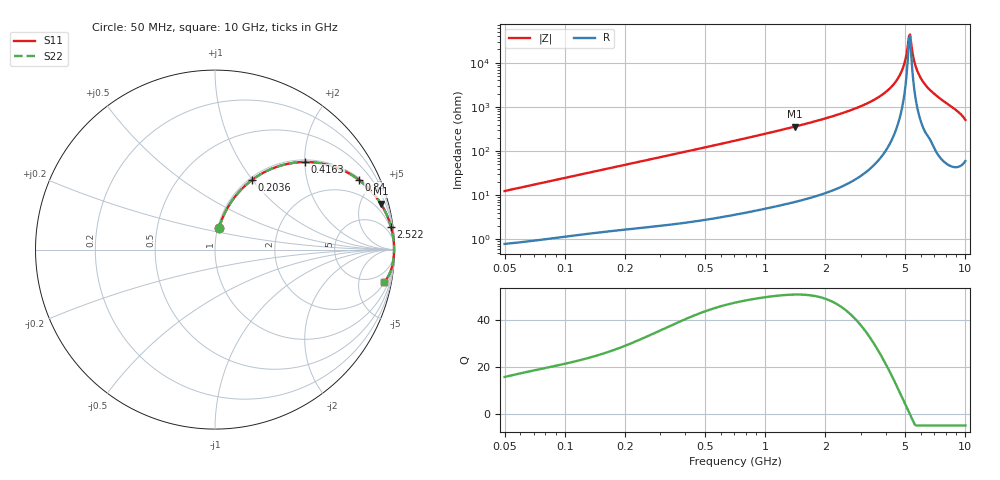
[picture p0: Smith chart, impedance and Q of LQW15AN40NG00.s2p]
!Murata Part Number: LQW15AN40NG00
!These Parameters are Measured in Series Mode Connection
!  o--[Z]--o
!Port1  Port2
!  o-------o
!Freq. Start=50[MHz] Stop=10[GHz], 401[Steps]
# Hz S RI R 50
!Freq.(Hz)	S 11(Real)	S 11(Imag)	S 21(Real)	S 21(Imag)	S 12(Real)	S 12(Imag)	S 22(Real)	S 22(Imag)
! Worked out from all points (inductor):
!   401 points, 50 MHz to 10 GHz, reference 50 ohm
!   read as one part in series: L = 39.4 nH near 51.34 MHz
!   highest Q = 51 at 1.408 GHz (marker M1), where L = 40.5 nH
!   self-resonance near 5.225 GHz
!   S11 on the Smith chart (normalised r, x): 50 MHz: 1.02, +0.25; 203.6 MHz: 1.03, +0.99; 416.3 MHz: 1.05, +2.01; 840 MHz: 1.08, +4.10; 2.522 GHz: 1, +15; 10 GHz: 2, -10
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5e7  0.0227 0.1205  0.9773 -0.1205  0.9773 -0.1205  0.0227 0.1205
1.214486e8  0.0909 0.2666  0.9091 -0.2666  0.9091 -0.2666  0.0909 0.2666
2.035837e8  0.2039 0.3862  0.7961 -0.3862  0.7961 -0.3862  0.2039 0.3862
2.949953e8  0.3409 0.4601  0.6591 -0.4601  0.6591 -0.4601  0.3409 0.4601
4.162766e8  0.5022 0.488  0.4978 -0.488  0.4978 -0.488  0.5022 0.488
7.071068e8  0.7424 0.4269  0.2576 -0.4269  0.2576 -0.4269  0.7424 0.4269
8.399791e8  0.8032 0.3875  0.1968 -0.3875  0.1968 -0.3875  0.8032 0.3875
1.408053e9  0.9235 0.2561  0.0765 -0.2561  0.0765 -0.2561  0.9235 0.2561
1.717543e9  0.9498 0.2087  0.0502 -0.2087  0.0502 -0.2087  0.9498 0.2087
2.521925e9  0.9805 0.1276  0.0195 -0.1276  0.0195 -0.1276  0.9805 0.1276
3.420121e9  0.9924 0.0722  0.00758 -0.0722  0.00758 -0.0722  0.9924 0.0722
4.171863e9  0.9964 0.0387  0.00363 -0.0387  0.00363 -0.0387  0.9964 0.0387
4.762728e9  0.9976 0.0168  0.00236 -0.0168  0.00236 -0.0168  0.9976 0.0168
4.955797e9  0.9978 0.0102  0.00218 -0.0102  0.00218 -0.0102  0.9978 0.0102
5.156693e9  0.9979 0.00359  0.00211 -0.00359  0.00211 -0.00359  0.9979 0.00359
5.295127e9  0.9979 -0.000862  0.00211 0.000862  0.00211 0.000862  0.9979 -0.000862
5.365732e9  0.9979 -0.0031  0.00213 0.0031  0.00213 0.0031  0.9979 -0.0031
5.583245e9  0.9977 -0.00986  0.00226 0.00986  0.00226 0.00986  0.9977 -0.00986
5.733131e9  0.9976 -0.0144  0.00242 0.0144  0.00242 0.0144  0.9976 -0.0144
6.207365e9  0.9966 -0.0285  0.00335 0.0285  0.00335 0.0285  0.9966 -0.0285
7.086521e9  0.9943 -0.0527  0.00571 0.0527  0.00571 0.0527  0.9943 -0.0527
1e10  0.9428 -0.1804  0.0572 0.1804  0.0572 0.1804  0.9428 -0.1804
